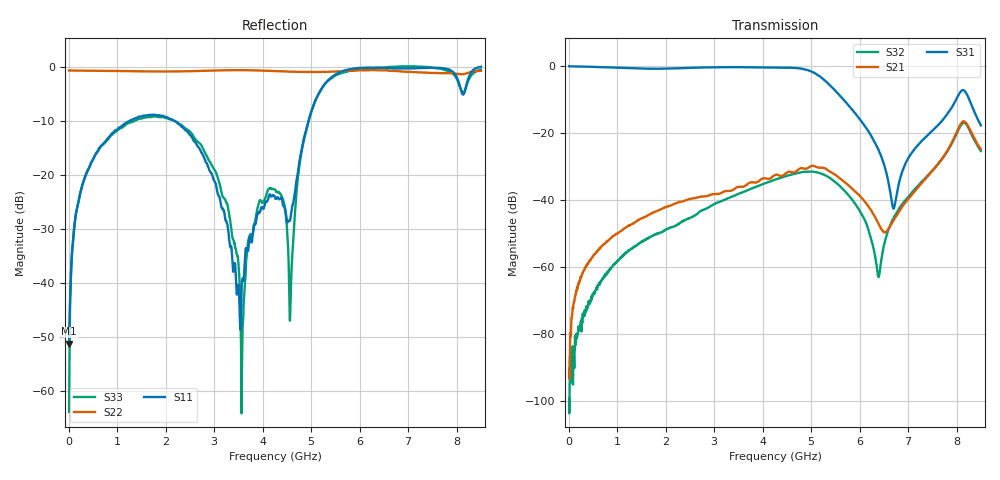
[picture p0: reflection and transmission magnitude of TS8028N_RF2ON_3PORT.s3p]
!Created with skrf (http://scikit-rf.org).
# GHz S RI R 50.0
!freq ReS11 ImS11 ReS12 ImS12 ReS13 ImS13
! ReS21 ImS21 ReS22 ImS22 ReS23 ImS23
! ReS31 ImS31 ReS32 ImS32 ReS33 ImS33
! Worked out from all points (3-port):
!   1601 points, 10 MHz to 8.5 GHz, reference 50 ohm
!   strongest paths, dB at 10 MHz, 2.132 GHz, 4.255 GHz, 6.378 GHz, 8.5 GHz:
!     S31: 0.0, -0.7, -0.4, -24.7, -17.7
!     S21: -90.2, -41.4, -32.5, -46.7, -24.8
!     S32: -99.4, -48.0, -33.9, -62.6, -25.4
!   lowest |S11| = -51.3 dB at 10 MHz (marker M1), VSWR 1.01, Z = 50.3 + j0.0276 ohm
!   |S11| at or under -10 dB: start of sweep to 1.263 GHz; 2.171 GHz to 4.948 GHz (2.777 GHz wide, 78 % of centre)
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0.01  0.00272 0.000274  7.41e-06 2.07e-05  0.9948 -0.00905
      -2.46e-06 3.07e-05  -0.9225 0.00532  -3.71e-06 1.18e-05
      0.9946 -0.00909  8.48e-06 -6.65e-06  0.000205 0.000605
0.1691875  0.00277 -0.048  -2.92e-05 0.000472  0.98 -0.0864
           -4.33e-05 0.000458  -0.9188 0.0551  -5.42e-05 -8.41e-05
           0.98 -0.0865  -4.82e-05 -8.7e-05  0.00329 -0.0488
0.9067563  -0.0962 -0.2244  -0.000447 0.00283  0.8566 -0.4075
           -0.000459 0.00281  -0.8768 0.2601  -0.00105 8.81e-05
           0.8564 -0.4076  -0.00103 0.000117  -0.1037 -0.2136
2.732106  -0.1444 -0.0732  0.002 0.011  0.2898 -0.9027
          0.00205 0.011  -0.5925 0.6975  -0.00424 0.00548
          0.29 -0.9033  -0.00423 0.00545  -0.1764 -0.0689
3.5758  0.00897 -0.00494  0.00414 0.0153  -0.2032 -0.9378
        0.00416 0.0152  -0.4551 0.8106  -0.00285 0.0127
        -0.2032 -0.9376  -0.00286 0.0127  0.00173 -0.000648
4.255  0.057 -0.023  0.0111 0.0209  -0.6377 -0.7051
       0.0112 0.0209  -0.3235 0.8526  0.00489 0.0195
       -0.6378 -0.7052  0.0049 0.0195  0.0441 -0.0581
4.573375  0.026 0.0297  0.017 0.0201  -0.8191 -0.467
          0.0171 0.0201  -0.2266 0.8704  0.0126 0.0201
          -0.8194 -0.4672  0.0126 0.0201  -0.00608 0.00167
5.082775  0.1012 0.4696  0.0299 0.0107  -0.7552 0.1797
          0.0299 0.0107  -0.0547 0.8904  0.0251 0.00763
          -0.7552 0.1794  0.0251 0.0077  0.2552 0.4107
6.393419  0.939 0.2703  0.00441 -0.000304  -0.013 0.0536
          0.00437 -0.000255  0.2152 0.9001  0.000601 0.000424
          -0.0131 0.0537  0.000587 0.000392  0.9708 -0.1259
8.5  0.8777 0.4793  0.0399 -0.0414  -0.0465 0.1214
     0.0397 -0.0414  0.6379 0.6575  0.0222 -0.0491
     -0.0466 0.1215  0.0223 -0.049  0.935 -0.1074
